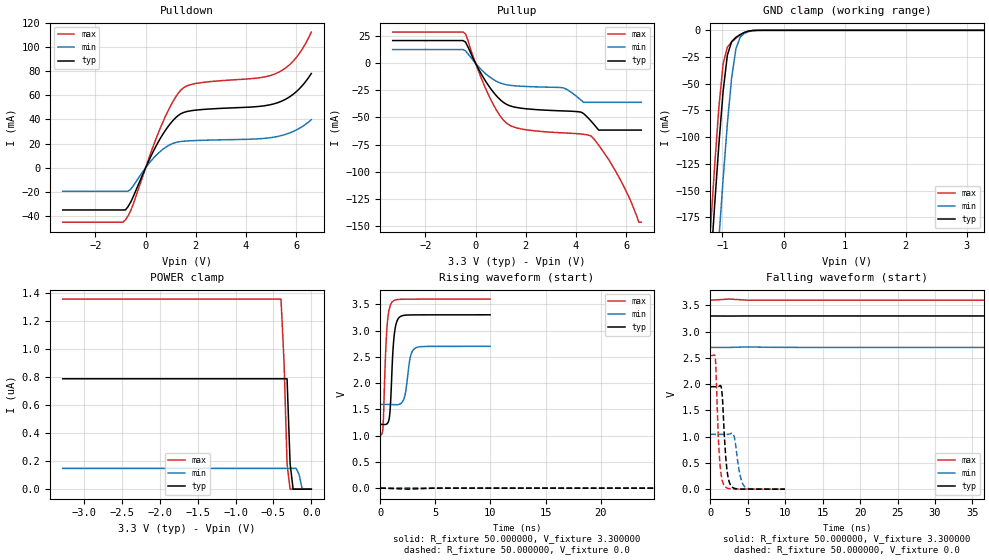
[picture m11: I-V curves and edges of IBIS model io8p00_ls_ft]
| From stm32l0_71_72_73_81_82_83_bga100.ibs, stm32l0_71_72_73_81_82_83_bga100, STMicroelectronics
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|   Model io8p00_ls_ft
[Model]  io8p00_ls_ft
Model_type I/O
Polarity   Non-Inverting
Enable   Active-Low
Vinl =   0.990000V
Vinh =   2.310000V
Vmeas =  1.650000V
Cref =   50.000000pF
Rref =   100.000000M
Vref =   0.0V
C_comp   4.606100pF   4.563500pF   4.706200pF
[Temperature Range]   25.000000   0.125000k   -40.000000
[Pullup Reference]   3.300000V   2.700000V   3.600000V
[Pulldown Reference]   0.0V   0.0V   0.0V
[POWER Clamp Reference]   3.300000V   2.700000V   3.600000V
[GND Clamp Reference]   0.0V   0.0V   0.0V
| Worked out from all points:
|   slope of the pulldown table from 0 to 0.495 V, typ, clamps not added: 23.6 ohm
|   slope of the pullup table from 0 to 0.495 V, typ, clamps not added: 24.9 ohm
|   GND clamp passes 1 mA (typ) near -0.59 V on its own axis
|   rising waveform, R_fixture 50.000000, V_fixture 3.300000: 20-80 % time 317ps typ, 427ps min, 299ps max; typ from 1.21 V to 3.3 V
|   rising waveform, R_fixture 50.000000, V_fixture 0.0: 20-80 % time 205ns typ, 424ns min, 100ns max; typ from 0 V to 1.95 V
|   falling waveform, R_fixture 50.000000, V_fixture 3.300000: 20-80 % time 194ns typ, 380ns min, 107ns max; typ from 3.3 V to 1.21 V
|   falling waveform, R_fixture 50.000000, V_fixture 0.0: 20-80 % time 520ps typ, 683ps min, 457ps max; typ from 1.95 V to 0 V
[Pulldown]
|Voltage   I(typ)   I(min)   I(max)
-3.3V     -34.78mA   -19.34mA   -44.89mA
-900mV    -34.78mA   -19.34mA   -44.89mA
-800mV    -34.78mA   -19.34mA   -42.84mA
-600mV    -28.56mA   -17.8mA    -35.75mA
100mV     4.638mA    2.744mA    6.076mA
600mV     24.8mA     13.84mA    33.52mA
1V        36.93mA    19.39mA    51.35mA
1.4V      44.67mA    21.76mA    64.17mA
2V        47.71mA    22.58mA    69.7mA
5.2V      53.44mA    25.71mA    78.05mA
6V        62.9mA     31.28mA    91.14mA
6.6V      77.96mA    39.76mA    112.2mA
[Pullup]
|Voltage   I(typ)   I(min)   I(max)
-3.3V     21.06mA    12.78mA    28.88mA
-400mV    19.65mA    11.53mA    27.22mA
400mV     -16.48mA   -9.566mA   -23.24mA
1.1V      -35.89mA   -19.06mA   -52.22mA
1.7V      -41.02mA   -20.95mA   -60.01mA
3.5V      -43.95mA   -22.7mA    -64.24mA
4.2V      -45.08mA   -33.97mA   -65.24mA
4.6V      -53.38mA   -36mA      -67.23mA
4.9V      -61.63mA   -36mA      -75.5mA
5.6V      -61.63mA   -36mA      -100.6mA
6.5V      -61.63mA   -36mA      -146.7mA
6.6V      -61.63mA   -36mA      -146.7mA
[GND_clamp]
|Voltage   I(typ)   I(min)   I(max)
-3.3V     -2.276A    -2.356A    -2.25A
-1.2V     -226mA     -318.7mA   -189.2mA
-1.13V    -164.9mA   -256.6mA   -128.3mA
-1.06V    -107.5mA   -196.5mA   -72.78mA
-990mV    -57.32mA   -139.4mA   -31.39mA
-920mV    -23.22mA   -87.32mA   -15.73mA
-850mV    -10.58mA   -44.45mA   -10.94mA
-780mV    -6.539mA   -17.25mA   -7.356mA
-710mV    -3.933mA   -6.349mA   -4.308mA
-640mV    -1.955mA   -2.79mA    -1.975mA
-360mV    -2.06uA    -16.21uA   -459.5nA
3.28V     0A         0A         0A
[POWER_clamp]
|Voltage   I(typ)   I(min)   I(max)
-3.28V    786.7nA    148nA      1.355uA
-400mV    786.7nA    148nA      1.355uA
-360mV    786.7nA    148nA      908.2nA
-320mV    786.7nA    148nA      180.5nA
-280mV    182.6nA    148nA      0A
-240mV    0A         148nA      0A
-200mV    0A         148nA      0A
-160mV    0A         101.6nA    0A
-120mV    0A         0A         0A
0V        0A         0A         0A
[Ramp]
| variable   typ   min   max
dV/dt_r  1.17105/0.20449u   0.60227/0.42541u   1.52766/99.97741n
dV/dt_f  1.25040/0.19362u   0.62460/0.37974u   1.55292/0.10674u
R_load = 50.000000
[Rising Waveform]
R_fixture= 50.000000
V_fixture= 3.300000
V_fixture_min= 2.700000
V_fixture_max= 3.600000
|time   V(typ)   V(min)   V(max)
0s        1.214V     1.593V     1.01V
240.2ps   1.212V     1.593V     1.142V
540.5ps   1.216V     1.593V     2.831V
800.8ps   1.313V     1.593V     3.394V
1.061ns   2.236V     1.592V     3.539V
1.341ns   3.03V      1.589V     3.58V
1.842ns   3.269V     1.607V     3.595V
2.222ns   3.291V     1.749V     3.596V
3.103ns   3.298V     2.656V     3.598V
9.97ns    3.3V       2.7V       3.599V
[Rising Waveform]
R_fixture= 50.000000
V_fixture= 0.0
V_fixture_min= 0.0
V_fixture_max= 0.0
|time   V(typ)   V(min)   V(max)
0s        47.89uV    15.54uV    94.67uV
47.55ns   443.7uV    -22.55uV   61.11mV
95.1ns    55.57mV    4.908uV    806.2mV
167.7ns   465.9mV    6.866mV    1.924V
210.2ns   771mV      18.04mV    2.275V
262.8ns   1.115V     60.97mV    2.452V
382.9ns   1.63V      227.1mV    2.533V
540.5ns   1.873V     500.6mV    2.545V
855.9ns   1.947V     887mV      2.546V
1.246us   1.952V     1.044V     2.546V
[Falling Waveform]
R_fixture= 50.000000
V_fixture= 3.300000
V_fixture_min= 2.700000
V_fixture_max= 3.600000
|time   V(typ)   V(min)   V(max)
0s        3.3V       2.7V       3.599V
82.58ns   3.3V       2.7V       3.499V
145.1ns   3.215V     2.7V       2.609V
217.7ns   2.823V     2.696V     1.582V
255.3ns   2.57V      2.685V     1.247V
292.8ns   2.308V     2.662V     1.117V
402.9ns   1.629V     2.54V      1.037V
515.5ns   1.353V     2.351V     1.019V
845.8ns   1.232V     1.789V     1.011V
1.246us   1.214V     1.593V     1.01V
[Falling Waveform]
R_fixture= 50.000000
V_fixture= 0.0
V_fixture_min= 0.0
V_fixture_max= 0.0
|time   V(typ)   V(min)   V(max)
0s        1.952V     1.044V     2.546V
680.7ps   1.952V     1.044V     2.483V
1.221ns   1.964V     1.044V     613.2mV
1.542ns   1.87V      1.044V     203.6mV
1.822ns   1.174V     1.044V     79.06mV
2.282ns   309mV      1.044V     18.38mV
2.903ns   42.56mV    1.066V     4.435mV
4.004ns   2.485mV    250.7mV    1.737mV
4.565ns   1.246mV    51.81mV    1.304mV
9.97ns    47.89uV    15.54uV    94.67uV
